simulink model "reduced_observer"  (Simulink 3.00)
settings: Solver=ode45  StartTime=0.0  StopTime=10.0  RelTol=1e-3
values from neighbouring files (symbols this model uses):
  A = [0 1 0 0;0 0 -mb*g/(1-mb) 0;0 0 0 1;0 0 m2_bar*g/(1-mb) 0]    [EXP7_2.M]    (also in EXP7_21.m; EXP6_10.M = [0 1 0;0 -1.799 6.953;0 0.939 -1.660]; EXP6_8.M = [a11 a12 0 -g;a21 a22 1 0;a31 a31 a33 0;0 1 0 0]; EXP6_9.m = [a11 a12 0 -g;a21 a22 1 0;a31 a31 a33 0;0 1 0 0])
  B = [0;1/((m+M)*(1-mb));0;-m2_bar/((m+M)*(1-mb))]    [EXP7_2.M]    (also in EXP7_21.m; EXP6_10.M = [0 0;-28.97 -6.453;-0.174 -0.230]; EXP6_8.M = [b1;b2;b3;0]; EXP6_9.m = [b1;b2;b3;0])
  C = [1 0 0 0;0 0 1 0]    [EXP7_2.M]    (also in EXP7_21.m; EXP6_8.M = [1 0 0 0]; EXP6_9.m = [1 0 0 0]; EXP7_1.M = [1 0 0 0])
  D = [-10 0;0 -10]    [EXP7_2.M]    (also in EXP7_21.m; EXP6_8.M = 0; Exp7_4.m)
  F1 = F(:,1:2)    [EXP7_2.M]    (also in EXP7_21.m; Exp7_4.m)
  F2 = F(:,3:4)    [EXP7_2.M]    (also in EXP7_21.m; Exp7_4.m)
  R = L*B    [EXP7_2.M]    (also in EXP7_21.m; Exp7_4.m; GAIN_CAL.M = B*inv(R2)*B')
  T = A12_taw+L_taw*A22_taw-D*L_taw    [EXP7_2.M]    (also in EXP7_21.m; Exp7_4.m)
libraries: simulink3 x8

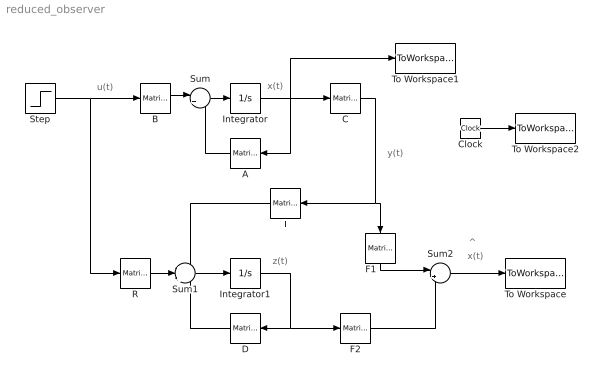
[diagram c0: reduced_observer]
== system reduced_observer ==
  note: u(t)
  note: x(t)
  note: y(t)
  note: z(t)
  note: x(t)
  note: ^
  A : simulink3/Math/Matrix Gain  Orientation=left  K=A
  B : simulink3/Math/Matrix Gain  K=B
  C : simulink3/Math/Matrix Gain  K=C
  Clock : Clock
  D : simulink3/Math/Matrix Gain  Orientation=left  K=D
  F1 : simulink3/Math/Matrix Gain  Orientation=down  K=F1
  F2 : simulink3/Math/Matrix Gain  K=F2
  Integrator : Integrator  ExternalReset=none  InitialConditionSource=internal  InitialCondition=[0.2 .1 -0.5 5]  LimitOutput=off  UpperSaturationLimit=inf  LowerSaturationLimit=-inf  ShowSaturationPort=off  ShowStatePort=off  AbsoluteTolerance=auto
  Integrator1 : Integrator  ExternalReset=none  InitialConditionSource=internal  InitialCondition=0  LimitOutput=off  UpperSaturationLimit=inf  LowerSaturationLimit=-inf  ShowSaturationPort=off  ShowStatePort=off  AbsoluteTolerance=auto
  R : simulink3/Math/Matrix Gain  K=R
  Step : Step  Time=0  Before=0  After=1  SampleTime=0
  Sum : Sum  Inputs=|++  SaturateOnIntegerOverflow=on
  Sum1 : Sum  Inputs=+++  SaturateOnIntegerOverflow=on
  Sum2 : Sum  Inputs=|++  SaturateOnIntegerOverflow=on
  T : simulink3/Math/Matrix Gain  Orientation=left  K=T
  To Workspace : ToWorkspace  VariableName=estim_state  SampleTime=-1  SaveFormat=Matrix
  To Workspace1 : ToWorkspace  VariableName=real_state  SampleTime=-1  SaveFormat=Matrix
  To Workspace2 : ToWorkspace  VariableName=time  SampleTime=-1  SaveFormat=Matrix
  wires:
  B/1 -> Sum/1
  Sum/1 -> Integrator/1
  Integrator/1 -> C/1, A/1, To Workspace1/1
  Sum1/1 -> Integrator1/1
  Step/1 -> B/1, R/1
  R/1 -> Sum1/2
  A/1 -> Sum/2
  D/1 -> Sum1/3
  T/1 -> Sum1/1
  Integrator1/1 -> D/1, F2/1
  F1/1 -> Sum2/1
  F2/1 -> Sum2/2
  Sum2/1 -> To Workspace/1
  Clock/1 -> To Workspace2/1
  C/1 -> F1/1, T/1
